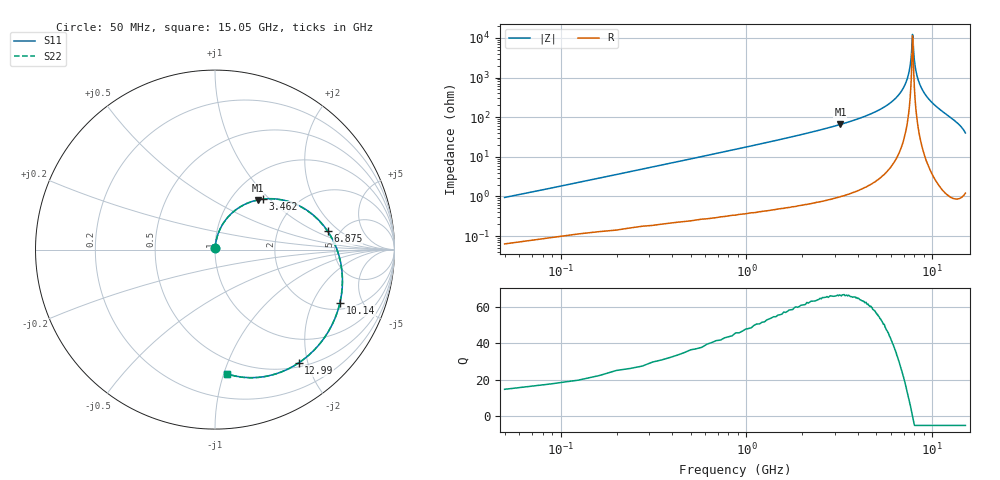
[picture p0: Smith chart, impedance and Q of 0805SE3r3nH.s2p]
! AVX Thin Film Operation		Date: May 2002
! Description: Accu-L® Series, Thin Film, SMD, RF Inductors
! Part Number: L08053R3CEWTR
! 50 MHz  -  15.05 GHz
! Serial Measurements
# mhz S db R 50
!	S11		S21		S12		S22
!	dB	Phase	dB	Phase	dB	Phase	dB	Phase
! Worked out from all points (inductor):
!   401 points, 50 MHz to 15.05 GHz, reference 50 ohm
!   read as 1/Y11, port 2 shorted: L = 2.86 nH near 125 MHz
!   highest Q = 66.5 at 3.2 GHz (marker M1), where L = 3.26 nH
!   self-resonance near 7.812 GHz
!   S11 on the Smith chart (normalised r, x): 50 MHz: 1.00, +0.01; 3.462 GHz: 1.38, +0.92; 6.875 GHz: 3.99, +1.38; 10.14 GHz: 2.36, -3.29; 12.99 GHz: 0.56, -1.85; 15.05 GHz: 0.38, -1.03
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50  -43.13 84.5  -0.01 -0.7  -0.01 -0.7  -43.13 84.5
162.5  -33.49 84.3  -0.01 -2.1  -0.01 -2.1  -33.49 84.3
275  -29.06 83.6  -0.02 -3.6  -0.02 -3.6  -29.06 83.6
462.5  -24.67 81.8  -0.04 -6.0  -0.04 -6.0  -24.67 81.7
687.5  -21.31 79.2  -0.06 -8.8  -0.06 -8.8  -21.31 79.2
1025  -17.95 75.3  -0.10 -13.1  -0.10 -13.1  -17.95 75.2
1437.5  -15.13 70.3  -0.17 -18.3  -0.17 -18.3  -15.13 70.3
1962.5  -12.58 64.0  -0.29 -24.8  -0.29 -24.8  -12.57 63.9
2562.5  -10.46 56.8  -0.46 -32.1  -0.46 -32.1  -10.46 56.7
3200  -8.77 49.4  -0.68 -39.7  -0.68 -39.7  -8.77 49.2
3462.5  -8.19 46.3  -0.78 -42.8  -0.78 -42.8  -8.19 46.2
5075  -5.61 28.3  -1.47 -61.0  -1.47 -61.0  -5.61 28.1
6875  -3.93 9.3  -2.35 -80.1  -2.35 -80.1  -3.93 9.1
7550  -3.49 2.5  -2.68 -87.0  -2.68 -87.0  -3.49 2.2
8825  -2.86 -10.2  -3.28 -99.7  -3.28 -99.7  -2.86 -10.5
10062.5  -2.44 -22.4  -3.80 -112.1  -3.80 -112.1  -2.44 -22.7
10137.5  -2.42 -23.2  -3.83 -112.8  -3.83 -112.8  -2.42 -23.5
11375  -2.17 -35.7  -4.21 -125.5  -4.21 -125.5  -2.17 -36.0
12575  -2.08 -48.7  -4.36 -138.7  -4.36 -138.7  -2.08 -49.0
12987.5  -2.11 -53.6  -4.34 -143.6  -4.34 -143.6  -2.11 -53.9
14150  -2.40 -69.0  -3.95 -159.4  -3.95 -159.4  -2.40 -69.3
15050  -3.15 -84.3  -3.17 -175.3  -3.17 -175.3  -3.16 -84.5
